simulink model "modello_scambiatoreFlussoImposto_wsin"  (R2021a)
settings: Solver=FixedStepAuto  StartTime=0.0  StopTime=100  FixedStep=0.05  RelTol=1e-3
undefined symbols (not defined in the file or in its folder): c, delta, K1, K2, m, Qeq, T0eq, tau, Tieq, weq

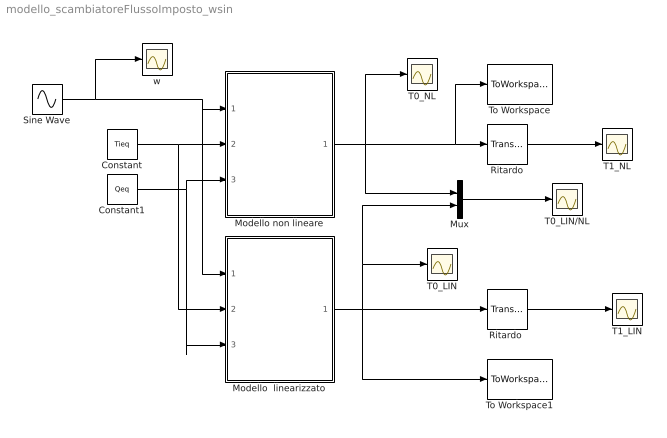
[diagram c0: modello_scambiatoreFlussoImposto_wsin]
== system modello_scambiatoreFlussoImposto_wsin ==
  Constant : Constant  Value=Tieq
  Constant1 : Constant  Value=Qeq
  Modello  linearizzato : Subsystem
  Modello non lineare : Subsystem
  Mux : Mux  Inputs=2
  Ritardo : TransportDelay  DelayTime=delta  InitialOutput=T0eq
  "Ritardo " : TransportDelay  DelayTime=delta  InitialOutput=T0eq
  Sine Wave : Sin  Amplitude=0.9*weq  Bias=weq  SampleTime=0
  T0_LIN : Scope
  T0_LIN/NL : Scope
  T0_NL : Scope
  T1_LIN : Scope
  T1_NL : Scope
  To Workspace : ToWorkspace  VariableName=T0NL  SaveFormat=Timeseries  SampleTime=-1
  To Workspace1 : ToWorkspace  VariableName=T0LIN  SaveFormat=Timeseries  SampleTime=-1
  w : Scope
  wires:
  Constant/1 -> Modello  linearizzato/2(Ti), Modello non lineare/2(Ti)
  Constant1/1 -> Modello  linearizzato/3(Q), Modello non lineare/3(Q)
  Modello non lineare/1(T0) -> Mux/1, T0_NL/1, Ritardo/1, To Workspace/1
  Ritardo/1 -> T1_NL/1
  Modello  linearizzato/1(T0) -> To Workspace1/1, T0_LIN/1, Mux/2, "Ritardo "/1
  "Ritardo "/1 -> T1_LIN/1
  Mux/1 -> T0_LIN/NL/1
  Sine Wave/1 -> w/1, Modello  linearizzato/1(w), Modello non lineare/1(w)

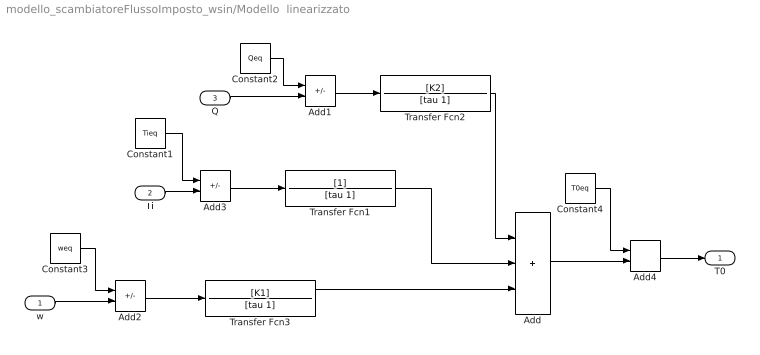
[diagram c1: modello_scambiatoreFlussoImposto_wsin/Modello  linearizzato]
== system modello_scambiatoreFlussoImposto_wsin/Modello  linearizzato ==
  w : Inport
  Ti : Inport  Port=2
  Q : Inport  Port=3
  Add : Sum  Inputs=+++
  Add1 : Sum  Inputs=-+
  Add2 : Sum  Inputs=-+
  Add3 : Sum  Inputs=-+
  Add4 : Sum
  Constant1 : Constant  Value=Tieq
  Constant2 : Constant  Value=Qeq
  Constant3 : Constant  Value=weq
  Constant4 : Constant  Value=T0eq
  Transfer Fcn1 : TransferFcn  Denominator=[tau 1]
  Transfer Fcn2 : TransferFcn  Numerator=[K2]  Denominator=[tau 1]
  Transfer Fcn3 : TransferFcn  Numerator=[K1]  Denominator=[tau 1]
  T0 : Outport
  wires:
  Add2/1 -> Transfer Fcn3/1
  w/1 -> Add2/2
  Constant3/1 -> Add2/1
  Transfer Fcn3/1 -> Add/3
  Ti/1 -> Add3/2
  Constant1/1 -> Add3/1
  Add3/1 -> Transfer Fcn1/1
  Transfer Fcn1/1 -> Add/2
  Q/1 -> Add1/2
  Constant2/1 -> Add1/1
  Add1/1 -> Transfer Fcn2/1
  Transfer Fcn2/1 -> Add/1
  Add/1 -> Add4/2
  Add4/1 -> T0/1
  Constant4/1 -> Add4/1

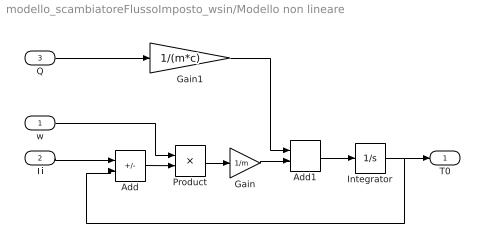
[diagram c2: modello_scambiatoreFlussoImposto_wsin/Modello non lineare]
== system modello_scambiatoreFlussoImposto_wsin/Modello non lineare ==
  w : Inport
  Ti : Inport  Port=2
  Q : Inport  Port=3
  Add : Sum  Inputs=+-
  Add1 : Sum
  Gain : Gain  Gain=1/m
  Gain1 : Gain  Gain=1/(m*c)
  Integrator : Integrator  InitialCondition=T0eq
  Product : Product
  T0 : Outport
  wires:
  Ti/1 -> Add/1
  Integrator/1 -> Add/2, T0/1
  Add/1 -> Product/2
  w/1 -> Product/1
  Product/1 -> Gain/1
  Gain/1 -> Add1/2
  Add1/1 -> Integrator/1
  Q/1 -> Gain1/1
  Gain1/1 -> Add1/1
